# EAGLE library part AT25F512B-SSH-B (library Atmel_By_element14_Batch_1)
Serial Flash Memory
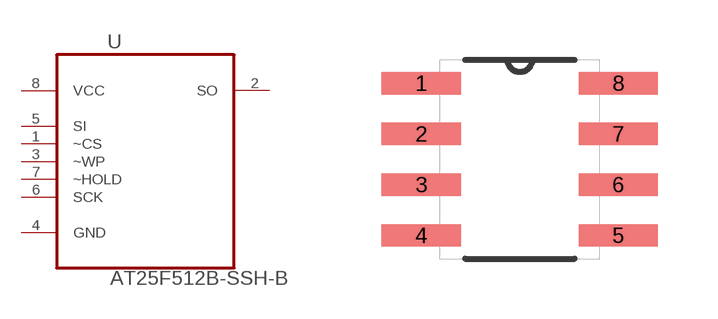
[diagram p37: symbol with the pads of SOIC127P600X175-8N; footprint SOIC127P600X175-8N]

Designator prefix U

## AT25F512B-SSH-B (MPN: AT25F512B-SSH-B; OC_FARNELL: 1715445; OC_NEWARK: 15R0311; PACKAGE: SOIC-8; SUPPLIER: Atmel)  [SOIC127P600X175-8N]
1  ~CS  in
2  SO  out
3  ~WP  in
4  GND  pas
5  SI  in
6  SCK  in
7  ~HOLD  in
8  VCC  pwr

## Footprint SOIC127P600X175-8N (pad centres in mm)
smd 1.981 x 0.559: 1 -2.464,1.905; 2 -2.464,0.635; 3 -2.464,-0.635; 4 -2.464,-1.905; 5 2.464,-1.905; 6 2.464,-0.635; 7 2.464,0.635; 8 2.464,1.905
